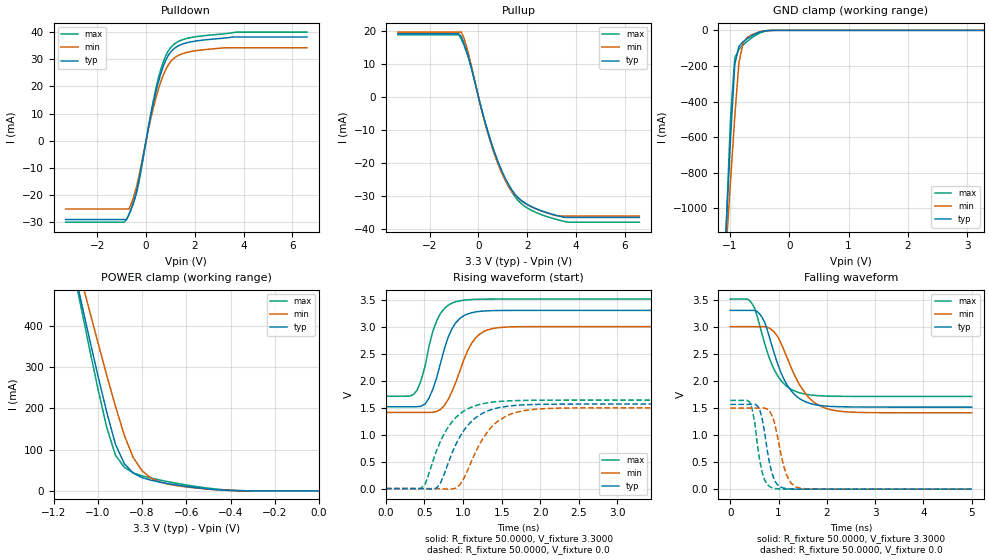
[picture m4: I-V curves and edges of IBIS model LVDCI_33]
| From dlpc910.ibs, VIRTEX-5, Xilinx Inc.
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|   Model LVDCI_33
[Model]  LVDCI_33
Model_type I/O
Polarity   Non-Inverting
Enable   Active-Low
Vinl = 0.76
Vinh = 2.2
Vmeas =  1.6500V
Cref =   0.0F
Rref =   1.0000M
Vref =   0.0V
C_comp   6.0000pF   6.0000pF   6.0000pF
[Model Spec]
Vinl   0.76   0.69   0.8
Vinh   2.2   2.0   2.3
[Temperature Range]   25.0000   85.0000   0.0
[Voltage Range]   3.3000V   3.0000V   3.4500V
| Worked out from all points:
|   slope of the pulldown table from 0 to 0.495 V, typ, clamps not added: 23.3 ohm
|   slope of the pullup table from 0 to 0.495 V, typ, clamps not added: 37.5 ohm
|   GND clamp passes 1 mA (typ) near -0.36 V on its own axis
|   POWER clamp passes 1 mA (typ) near -0.40 V on its own axis
|   rising waveform, R_fixture 50.0000, V_fixture 3.3000: 20-80 % time 235ps typ, 274ps min, 204ps max; typ from 1.51 V to 3.3 V
|   rising waveform, R_fixture 50.0000, V_fixture 0.0: 20-80 % time 347ps typ, 362ps min, 334ps max; typ from 0 V to 1.56 V
|   falling waveform, R_fixture 50.0000, V_fixture 3.3000: 20-80 % time 450ps typ, 533ps min, 428ps max; typ from 3.3 V to 1.51 V
|   falling waveform, R_fixture 50.0000, V_fixture 0.0: 20-80 % time 187ps typ, 229ps min, 167ps max; typ from 1.56 V to 0 V
[Pulldown]
|Voltage   I(typ)   I(min)   I(max)
-3.3V     -29.02mA   -25.15mA   -30mA
-800mV    -29.02mA   -25.15mA   -28.94mA
-700mV    -27.16mA   -25.15mA   -27.13mA
-400mV    -19.09mA   -17.25mA   -19.55mA
-200mV    -10.05mA   -8.934mA   -10.66mA
200mV     9.61mA     8.407mA    10.29mA
600mV     24.61mA    21.63mA    26.16mA
900mV     31.25mA    27.76mA    32.92mA
1.2V      34.29mA    30.76mA    35.91mA
2V        36.68mA    33.11mA    38.26mA
3.7V      38.22mA    34.24mA    40.02mA
6.6V      38.22mA    34.24mA    40.02mA
[Pullup]
|Voltage   I(typ)   I(min)   I(max)
-3.3V     19.05mA    19.57mA    18.76mA
-800mV    19.05mA    19.57mA    18.76mA
-700mV    18.13mA    19.57mA    17.42mA
-600mV    16.29mA    17.88mA    15.7mA
-400mV    11.84mA    12.79mA    11.57mA
200mV     -5.757mA   -6.028mA   -5.78mA
700mV     -17.69mA   -18.34mA   -17.86mA
1.2V      -26.14mA   -26.73mA   -26.63mA
1.7V      -31.1mA    -31.25mA   -32.06mA
2.6V      -34.65mA   -34.71mA   -35.82mA
3.6V      -36.63mA   -36.21mA   -37.96mA
6.6V      -36.63mA   -36.21mA   -38.06mA
[GND_clamp]
|Voltage   I(typ)   I(min)   I(max)
-3.3V     -16.97A    -12.88A    -20.48A
-1.13V    -1.567A    -1.562A    -1.656A
-1.06V    -1.075A    -1.198A    -1.059A
-990mV    -594.4mA   -837.2mA   -482.9mA
-920mV    -191.9mA   -483.2mA   -155.6mA
-850mV    -89.88mA   -181.4mA   -105.9mA
-780mV    -63.96mA   -70.51mA   -82.33mA
-710mV    -46.62mA   -40.81mA   -61.99mA
-640mV    -31.71mA   -26.56mA   -43.7mA
-500mV    -9.786mA   -8.389mA   -15.42mA
-290mV    -155.5uA   -193.9uA   -401.9uA
3.28V     28.06nA    90.59uA    57.71nA
[POWER_clamp]
|Voltage   I(typ)   I(min)   I(max)
-3.28V    5.82A      5.011A     6.424A
-1.12V    567.4mA    604.5mA    564.7mA
-1.08V    470.7mA    523.2mA    456.9mA
-1.04V    374.3mA    442mA      351.1mA
-960mV    191.7mA    281.1mA    154.6mA
-920mV    112.8mA    204.8mA    86.55mA
-880mV    65.86mA    134.5mA    56.98mA
-840mV    43.25mA    81.04mA    43.8mA
-760mV    26.01mA    31.15mA    31.13mA
-680mV    17.61mA    16.23mA    22.15mA
-400mV    1.02mA     1.137mA    1.723mA
0V        29.68nA    137.7nA    65.13nA
[Ramp]
| variable   typ   min   max
dV/dt_r  0.9390/0.3465n   0.8970/0.3596n   0.9828/0.3325n
dV/dt_f  1.0710/0.4491n   0.9540/0.5316n   1.1238/0.4202n
R_load = 50.0000
[Rising Waveform]
R_fixture= 50.0000
V_fixture= 3.3000
V_fixture_min= 3.0000
V_fixture_max= 3.6000
|time   V(typ)   V(min)   V(max)
0s        1.515V     1.41V      1.711V
350ps     1.515V     1.41V      1.733V
450ps     1.523V     1.41V      1.973V
510ps     1.567V     1.41V      2.279V
660ps     2.063V     1.428V     3.113V
810ps     2.813V     1.656V     3.397V
910ps     3.078V     1.984V     3.461V
1.11ns    3.256V     2.688V     3.5V
1.41ns    3.296V     2.97V      3.509V
5ns       3.3V       2.999V     3.509V
[Rising Waveform]
R_fixture= 50.0000
V_fixture= 0.0
|time   V(typ)   V(min)   V(max)
0s        814.7nV    1.06uV     1.855uV
450ps     -1.205mV   -2.76uV    -777.4uV
510ps     -4.242mV   35.63uV    82.57mV
660ps     12.56mV    -2.074mV   714.5mV
810ps     480.2mV    -10.02mV   1.145V
960ps     963.7mV    72.48mV    1.384V
1.26ns    1.4V       934.9mV    1.572V
1.52ns    1.512V     1.31V      1.617V
1.87ns    1.554V     1.459V     1.634V
5ns       1.565V     1.495V     1.638V
[Falling Waveform]
R_fixture= 50.0000
V_fixture= 3.3000
V_fixture_min= 3.0000
V_fixture_max= 3.6000
|time   V(typ)   V(min)   V(max)
0s        3.3V       3V         3.509V
400ps     3.3V       3V         3.485V
610ps     3.233V     3V         3.022V
710ps     3.084V     2.999V     2.696V
960ps     2.369V     2.845V     2.124V
1.16ns    1.95V      2.464V     1.906V
1.36ns    1.723V     2.053V     1.801V
1.67ns    1.578V     1.653V     1.738V
2.12ns    1.526V     1.46V      1.716V
5ns       1.515V     1.41V      1.711V
[Falling Waveform]
R_fixture= 50.0000
V_fixture= 0.0
|time   V(typ)   V(min)   V(max)
0s        1.565V     1.495V     1.638V
400ps     1.565V     1.495V     1.609V
510ps     1.567V     1.495V     1.213V
560ps     1.54V      1.495V     835.5mV
710ps     1.051V     1.496V     174.8mV
860ps     305.4mV    1.369V     27.17mV
960ps     100.6mV    1.051V     8.006mV
1.16ns    10.66mV    276mV      857uV
1.36ns    1.378mV    43.58mV    133.8uV
5ns       9.855uV    40.87uV    30.34uV
